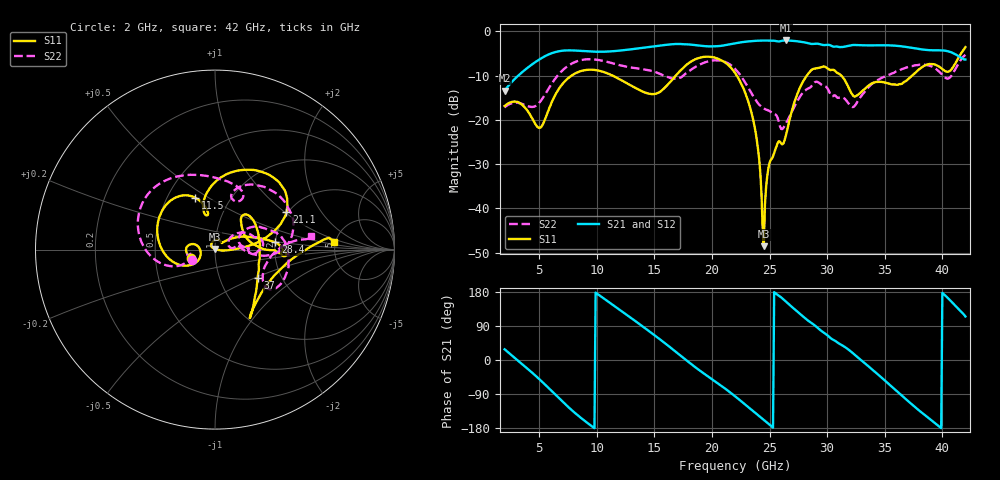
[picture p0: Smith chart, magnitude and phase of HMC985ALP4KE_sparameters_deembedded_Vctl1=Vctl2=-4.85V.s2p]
!s2p File: Measurements: S11, S21, S12, S22
# GHz S dB R 50.0
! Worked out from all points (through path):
!   401 points, 2 GHz to 42 GHz, reference 50 ohm
!   highest |S21| = -2.06 dB at 26.4 GHz (marker M1); lowest = -13.4 dB at 2 GHz (marker M2)
!   lowest |S11| = -48.5 dB at 24.5 GHz (marker M3), VSWR 1.01, Z = 49.9 + j0.349 ohm
!   |S11| at or under -10 dB: start of sweep to 7.813 GHz; 22.16 GHz to 28.23 GHz (6.079 GHz wide, 24.1 % of centre); 31.23 GHz to 37.38 GHz (6.148 GHz wide, 17.9 % of centre)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
!   |S22| runs from -22.1 to -5.3 dB; largest |S21 - S12| = 0.001
!   S11 on the Smith chart (normalised r, x): 2 GHz: 0.76, -0.07; 11.5 GHz: 0.69, +0.44; 21.1 GHz: 1.97, +1.02; 28.4 GHz: 2.00, +0.18; 37 GHz: 1.51, -0.52; 42 GHz: 4.80, +0.77
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2  -16.87 -161.8  -13.43 28.2  -13.43 28.3  -17.17 -155.6
5  -21.82 -172.6  -6.37 -50.1  -6.38 -50.1  -16.16 -159.8
6.3  -14.85 -150.3  -4.76 -88.3  -4.76 -88.3  -11.02 -161.6
8.7  -8.92 150.3  -4.44 -154.6  -4.44 -154.6  -6.46 151.2
11.5  -10.17 111.1  -4.47 143.1  -4.47 143.1  -7.31 105.0
13.6  -13.12 101.2  -3.85 97.1  -3.85 97.1  -8.40 75.6
15.4  -13.81 105.9  -3.25 56.4  -3.25 56.4  -9.51 62.0
17.9  -7.33 80.2  -2.94 -3.6  -2.94 -3.5  -9.20 72.0
21.1  -6.96 27.6  -3.14 -74.4  -3.15 -74.4  -6.86 16.0
22  -9.35 17.0  -2.71 -95.6  -2.71 -95.6  -8.46 0.5
23.6  -20.24 0.1  -2.18 -135.3  -2.17 -135.3  -14.73 -4.5
24.5  -48.53 110.7  -2.08 -158.0  -2.08 -157.9  -17.41 8.1
25  -29.68 132.0  -2.10 -170.7  -2.10 -170.7  -18.00 10.9
26.4  -23.70 41.5  -2.06 154.6  -2.06 154.6  -20.93 32.7
28.4  -9.42 6.8  -2.71 102.6  -2.71 102.7  -12.86 18.2
28.7  -8.59 1.9  -2.85 96.4  -2.85 96.4  -12.18 16.3
30.7  -8.96 -3.1  -3.44 50.5  -3.44 50.5  -14.48 2.0
32.5  -14.62 31.6  -3.09 10.8  -3.09 10.8  -16.45 27.5
35.4  -11.81 19.2  -3.16 -64.7  -3.16 -64.7  -9.79 19.3
37  -10.88 -33.7  -3.58 -107.8  -3.58 -107.8  -8.06 4.9
39.8  -8.11 -57.5  -4.29 -177.4  -4.29 -177.3  -9.29 -36.0
42  -3.57 3.9  -6.35 114.9  -6.36 114.9  -5.32 8.3
